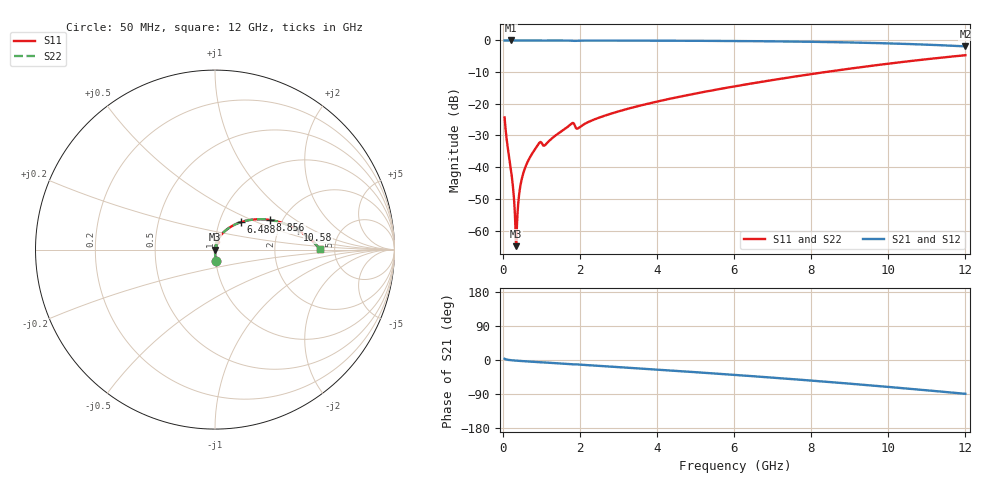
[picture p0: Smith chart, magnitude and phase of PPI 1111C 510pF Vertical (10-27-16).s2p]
# GHz S MA R 50
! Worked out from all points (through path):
!   1601 points, 50 MHz to 12 GHz, reference 50 ohm
!   highest |S21| = 0.00 dB at 206.8 MHz (marker M1); lowest = -1.9 dB at 12 GHz (marker M2)
!   group delay of S21, straight-line fit = 20.5 ps
!   lowest |S11| = -64.9 dB at 348.8 MHz (marker M3), VSWR 1.00, Z = 50.1 - j0.00194 ohm
!   |S11| at or under -10 dB: start of sweep to 8.357 GHz
!   |S22| runs from -64.9 to -4.7 dB; largest |S21 - S12| = 0
!   S11 on the Smith chart (normalised r, x): 50 MHz: 1.00, -0.12; 6.488 GHz: 1.27, +0.41; 8.856 GHz: 1.73, +0.65; 10.58 GHz: 2.56, +0.72; 12 GHz: 3.81, +0.04
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0.05  0.06096 -86.5  0.9979 3.3  0.9979 3.3  0.06096 -86.5
0.2068437  0.009802 -87.8  0.9995 -0.4  0.9995 -0.4  0.009802 -87.8
0.259125  0.005432 -85.6  0.9995 -0.9  0.9995 -0.9  0.005432 -85.6
0.3114062  0.002112 -76.6  0.9994 -1.4  0.9994 -1.4  0.002112 -76.6
0.34875  0.0005667 -2.0  0.9994 -1.7  0.9994 -1.7  0.0005667 -2.0
0.3860938  0.001927 70.1  0.9994 -2.0  0.9994 -2.0  0.001927 70.1
0.4533125  0.004836 80.0  0.9993 -2.5  0.9993 -2.5  0.004836 80.0
0.5429375  0.008351 82.1  0.9992 -3.1  0.9992 -3.1  0.008351 82.1
0.677375  0.01323 82.4  0.9991 -4.0  0.9991 -4.0  0.01323 82.4
0.9014375  0.02199 78.9  0.9976 -5.6  0.9976 -5.6  0.02199 78.9
1.110562  0.02264 74.7  0.9963 -6.7  0.9963 -6.7  0.02264 74.7
1.78275  0.0485 71.5  0.9928 -11.4  0.9928 -11.4  0.0485 71.5
1.939594  0.04052 67.8  0.9916 -11.7  0.9916 -11.7  0.04052 67.8
2.044156  0.0449 73.4  0.9956 -12.5  0.9956 -12.5  0.0449 73.4
4.038312  0.1096 63.4  0.9919 -25.6  0.9919 -25.6  0.1096 63.4
6.025  0.189 49.9  0.9793 -39.4  0.9793 -39.4  0.189 49.9
6.488062  0.2111 46.6  0.9746 -42.7  0.9746 -42.7  0.2111 46.6
8.019156  0.2953 35.0  0.952 -54.4  0.952 -54.4  0.2953 35.0
8.855656  0.3487 28.2  0.9334 -61.2  0.9334 -61.2  0.3487 28.2
10.01331  0.4307 18.4  0.8982 -71.1  0.8982 -71.1  0.4307 18.4
10.58094  0.4735 13.3  0.8762 -76.2  0.8762 -76.2  0.4735 13.3
12  0.5844 0.3  0.8062 -89.2  0.8062 -89.2  0.5844 0.3
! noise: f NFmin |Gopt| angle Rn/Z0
0.05  0.0003603  0.862  0.2816  0.0005595
1.372  0.004545  0.7229  6.555  0.003243
2.701  0.006661  0.647  12.67  0.003537
4.031  0.008593  0.607  18.52  0.003946
5.36  0.01068  0.5913  24.15  0.004593
6.682  0.01284  0.5869  29.53  0.005334
8.012  0.01515  0.5907  34.7  0.006215
9.341  0.01767  0.6014  39.67  0.007291
10.67  0.0205  0.6181  44.46  0.008646
12  0.02375  0.6398  49.12  0.0104
